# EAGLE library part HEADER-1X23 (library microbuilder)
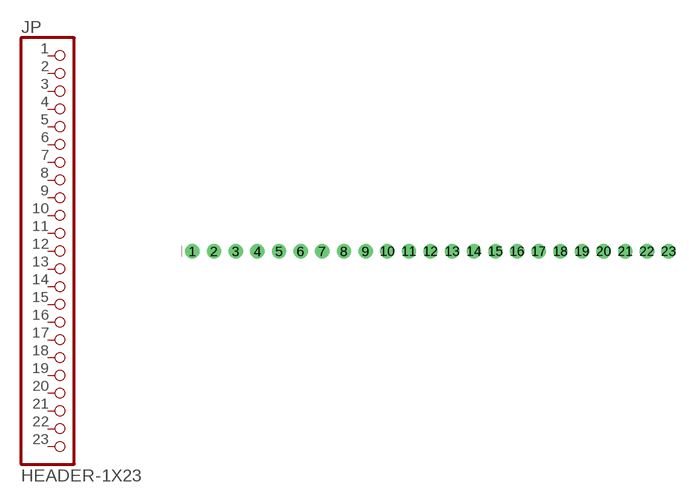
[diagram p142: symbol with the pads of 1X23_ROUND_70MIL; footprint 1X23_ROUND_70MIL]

Designator prefix JP

## HEADER-1X23  [1X23_ROUND_70MIL]
1  1  pas
2  2  pas
3  3  pas
4  4  pas
5  5  pas
6  6  pas
7  7  pas
8  8  pas
9  9  pas
10  10  pas
11  11  pas
12  12  pas
13  13  pas
14  14  pas
15  15  pas
16  16  pas
17  17  pas
18  18  pas
19  19  pas
20  20  pas
21  21  pas
22  22  pas
23  23  pas

## Footprint 1X23_ROUND_70MIL (pad centres in mm)
drill 1 pad 1.676: 1 -27.94,0; 2 -25.4,0; 3 -22.86,0; 4 -20.32,0; 5 -17.78,0; 6 -15.24,0; 7 -12.7,0; 8 -10.16,0; 9 -7.62,0; 10 -5.08,0; 11 -2.54,0; 12 0,0; 13 2.54,0; 14 5.08,0; 15 7.62,0; 16 10.16,0; 17 12.7,0; 18 15.24,0; 19 17.78,0; 20 20.32,0; 21 22.86,0; 22 25.4,0; 23 27.94,0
